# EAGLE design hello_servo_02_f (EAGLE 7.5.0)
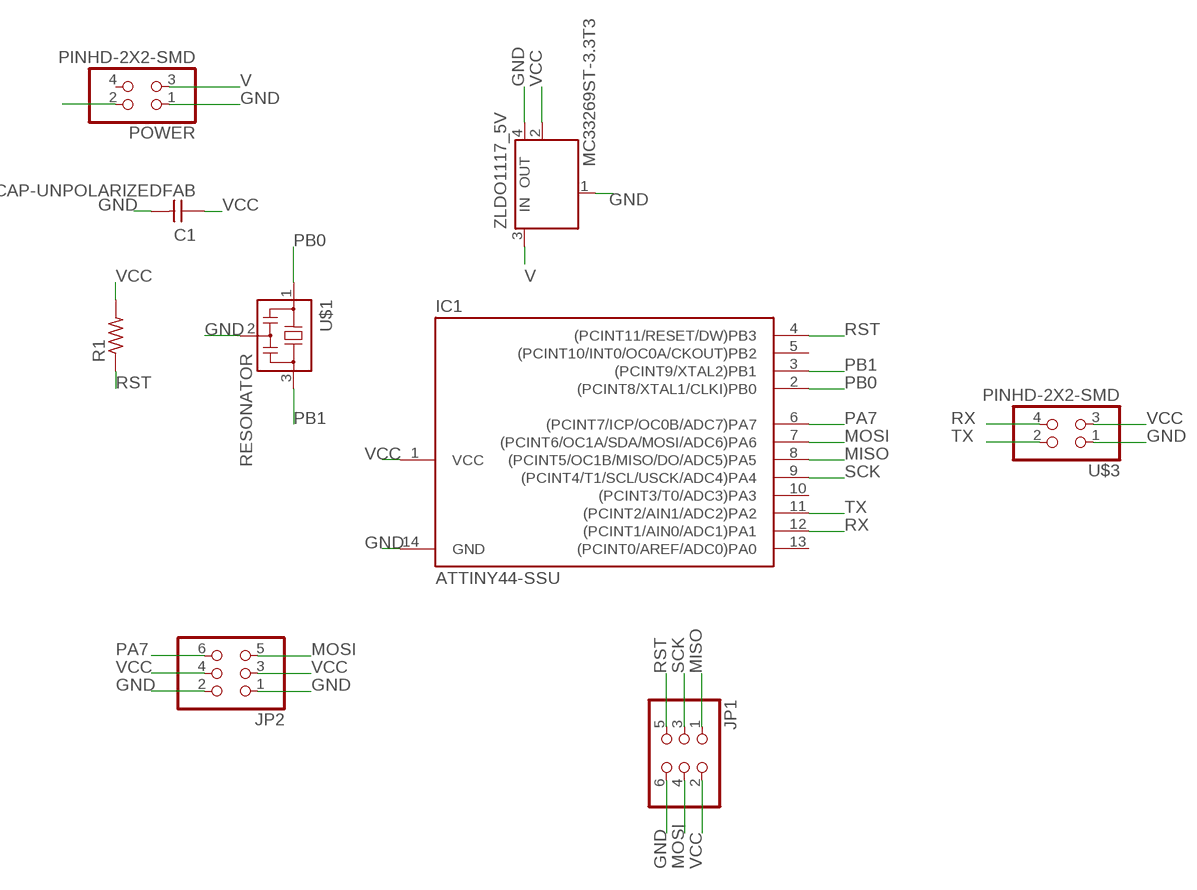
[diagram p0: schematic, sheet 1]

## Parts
C1  CAP-UNPOLARIZEDFAB  [C1206FAB]
IC1  ATTINY44-SSU  [SOIC14]
JP1  PINHD-2X3-SMD  [2X03SMD]
JP2  PINHD-2X3-SMD  [2X03SMD]
POWER  PINHD-2X2-SMD  [2X02SMD]
R1  RES-US1206FAB  [R1206FAB]
U$1  RESONATOR  [EFOBM]
U$3  PINHD-2X2-SMD  [2X02SMD]
ZLDO1117_5V  MC33269ST-3.3T3  [SOT223]

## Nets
GND: C1.2 IC1.14(GND) JP1.6 JP2.1 JP2.2 POWER.1 POWER.2 U$1.2 U$3.1 ZLDO1117_5V.1(GND/ADJ) ZLDO1117_5V.4(OUT)
MISO: IC1.8((PCINT5/OC1B/MISO/DO/ADC5)PA5) JP1.1
MOSI: IC1.7((PCINT6/OC1A/SDA/MOSI/ADC6)PA6) JP1.4 JP2.5
PA7: IC1.6((PCINT7/ICP/OC0B/ADC7)PA7) JP2.6
PB0: IC1.2((PCINT8/XTAL1/CLKI)PB0) U$1.1
PB1: IC1.3((PCINT9/XTAL2)PB1) U$1.3
RST: IC1.4((PCINT11/RESET/DW)PB3) JP1.5 R1.1
RX: IC1.12((PCINT1/AIN0/ADC1)PA1) U$3.4
SCK: IC1.9((PCINT4/T1/SCL/USCK/ADC4)PA4) JP1.3
TX: IC1.11((PCINT2/AIN1/ADC2)PA2) U$3.2
V: POWER.3 ZLDO1117_5V.3(IN)
VCC: C1.1 IC1.1(VCC) JP1.2 JP2.3 JP2.4 R1.2 U$3.3 ZLDO1117_5V.2(OUT)
Unconnected: IC1.5((PCINT10/INT0/OC0A/CKOUT)PB2) IC1.10((PCINT3/T0/ADC3)PA3) IC1.13((PCINT0/AREF/ADC0)PA0) POWER.4

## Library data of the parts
C1 = fab:CAP-UNPOLARIZED
IC1 = fab:ATTINY44
JP1 JP2 = fab:PINHD-2X3-SMD: PIN HEADER
POWER U$3 = fab:PINHD-2X2-SMD
R1 = fab:RES-US: Resistor (US Symbol)
U$1 = fab:RESONATOR
ZLDO1117_5V = linear:MC33269ST*: Adjustable Output Low Dropout Voltage Regulator 800 mA Source: http://www.onsemi.com/pub/Collateral/MC33269-D.PDF

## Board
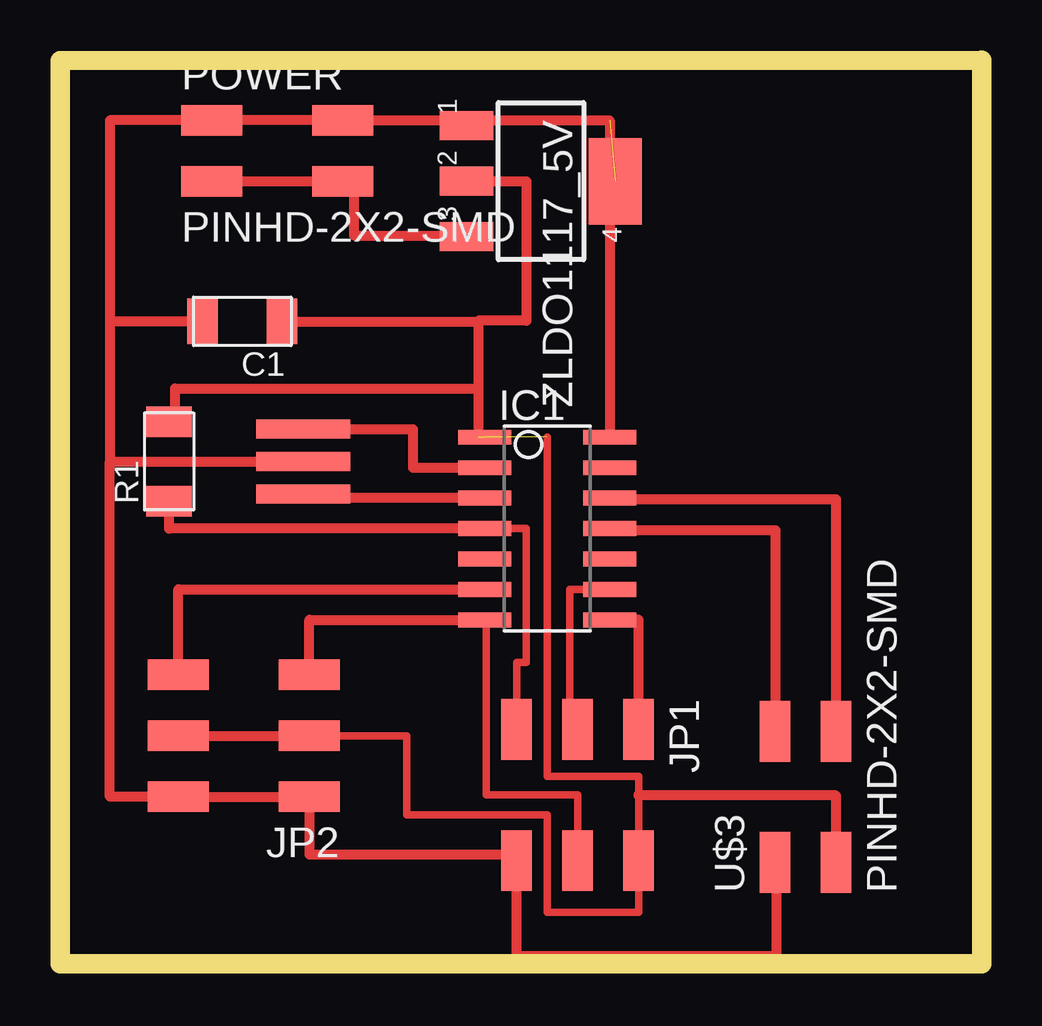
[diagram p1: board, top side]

Size 38.41 x 37.67 mm. Coordinates in mm from the lower left corner, seen from the top.
Outline: 0,0 38.41,0 38.41,37.67 0,37.64 0,0
Copper layers (1*16): Top 0.035mm / dielectric 1.5mm / Bottom 0.035mm
Design rules "default": minimum track width 10mil, minimum drill 24mil, track to track 8mil, track to pad 8mil, pad to pad 8mil, via to via 8mil, smd to smd 8mil, copper to edge 40mil, drill to drill 8mil, minimum pad ring 10mil, minimum via ring 8mil, stop-mask expansion 4mil, vias tented up to drill 0mil, thermal gap 10mil

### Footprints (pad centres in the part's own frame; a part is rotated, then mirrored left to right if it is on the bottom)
C1206FAB = smd 1.27 x 1.905: 1 -1.651,0; 2 1.651,0
SOIC14 = smd 0.61 x 2.21: 1 -3.81,-2.603; 2 -2.54,-2.603; 3 -1.27,-2.603; 4 0,-2.603; 5 1.27,-2.603; 6 2.54,-2.603; 7 3.81,-2.603; 8 3.81,2.603; 9 2.54,2.603; 10 1.27,2.603; 11 0,2.603; 12 -1.27,2.603; 13 -2.54,2.603; 14 -3.81,2.603
2X03SMD = smd 2.54 x 1.27: 1 -2.54,2.54; 2 2.92,2.54; 3 -2.54,0; 4 2.92,0; 5 -2.54,-2.54; 6 2.92,-2.54
2X02SMD = smd 2.54 x 1.27: 1 -2.54,1.27; 2 2.92,1.27; 3 -2.54,-1.27; 4 2.92,-1.27
R1206FAB = smd 1.27 x 1.905: 1 -1.651,0; 2 1.651,0
EFOBM = smd 0.8 x 3.9: 1 -1.35,0; 2 0,0; 3 1.35,0
SOT223 = smd 1.219 x 2.235: 1 -2.311,-3.099; 2 0,-3.099; 3 2.311,-3.099 | smd 3.6 x 2.2: 4 0,3.099

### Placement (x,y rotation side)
C1  7.59,26.77 180 top
IC1  20.29,18.14 270 top
JP1  21.56,7.21 270 top
JP2  7.85,9.5 180 top
POWER  8.86,33.88 0 top
R1  4.55,20.93 90 top
U$1  10.13,20.93 270 top
U$3  31.06,6.76 90 top
ZLDO1117_5V  20.04,32.61 270 top

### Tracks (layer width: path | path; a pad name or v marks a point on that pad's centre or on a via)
GND  (1 unrouted)
  Top 0.406: 2.08,20.93 U$1.2 | 2.08,20.93 2.08,6.96 JP2.2 JP2.1 10.39,4.55 19.02,4.55 JP1.6 19.02,0.3 29.84,0.3 29.84,4.22 U$3.1 | 2.08,26.77 2.08,20.93 | C1.2 2.08,26.77 | 16.94,35.15 ZLDO1117_5V.1 17.09,34.92 17.09,34.62 16.69,34.62 16.69,35.15 | POWER.1 2.08,35.15 2.08,26.77 | 6.32,34.92 POWER.1 | 16.69,35.15 POWER.2 POWER.1 | 16.69,35.15 22.9,35.15 IC1.14
MISO
  Top 0.406: JP1.1 24.1,14.33 IC1.8
MOSI
  Top 0.305: 17.75,14.33 17.75,7.04 21.56,7.04 JP1.4
  Top 0.406: 17.75,14.33 IC1.7 10.39,14.33 JP2.5
PA7
  Top 0.406: JP2.6 4.93,15.6 IC1.6
PB0
  Top 0.406: U$1.1 14.71,22.28 14.71,20.68 IC1.2
PB1
  Top 0.406: IC1.3 10.13,19.41 U$1.3
RST
  Top 0.305: IC1.4 19.43,18.14 19.43,12.55 19.02,12.55 JP1.5
  Top 0.406: IC1.4 4.55,18.14 R1.1
RX
  Top 0.406: U$3.4 32.33,19.35 22.9,19.35 IC1.12
SCK
  Top 0.305: 21.23,9.75 21.23,15.6 IC1.9
  Top 0.406: JP1.3 21.23,9.75
TX
  Top 0.406: U$3.2 29.82,9.68 29.82,18.06 22.9,18.06 IC1.11
V
  Top 0.406: POWER.3 11.86,32.61 11.86,32.84 12.24,32.84 12.24,30.35 16.94,30.35 ZLDO1117_5V.3
VCC  (2 unrouted)
  Top 0.305: JP2.3 14.45,9.5 14.45,6.2 20.29,6.2 20.29,2.13 24.1,2.13 JP1.2 24.1,7.04 24.1,7.8 20.29,7.8 20.29,21.95
  Top 0.406: R1.2 4.8,22.58 4.8,23.98 17.44,23.98 | 17.44,23.98 17.44,21.95 | JP2.4 JP2.3 | C1.1 17.44,26.77 | 17.44,26.77 17.44,23.98 | U$3.3 32.33,7.01 24.1,7.01 24.1,7.04 | ZLDO1117_5V.2 19.43,32.61 19.43,26.8 17.44,26.8 17.44,26.77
